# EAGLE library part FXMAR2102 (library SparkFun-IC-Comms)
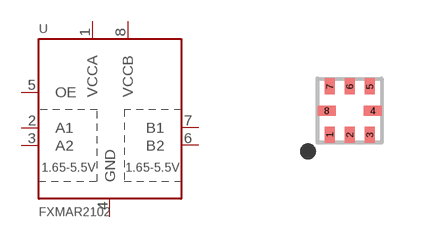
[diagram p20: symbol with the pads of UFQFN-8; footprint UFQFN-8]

Designator prefix U

## FXMAR2102  [UFQFN-8]
1  VCCA
2  A1
3  A2
4  GND
5  OE
6  B2
7  B1
8  VCCB

## Footprint UFQFN-8 (pad centres in mm)
smd 0.25 x 0.4: 1 -0.5,-0.605; 2 0,-0.605; 3 0.5,-0.605; 5 0.5,0.605; 6 0,0.605; 7 -0.5,0.605
smd 0.45 x 0.25: 4 0.575,0; 8 -0.575,0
